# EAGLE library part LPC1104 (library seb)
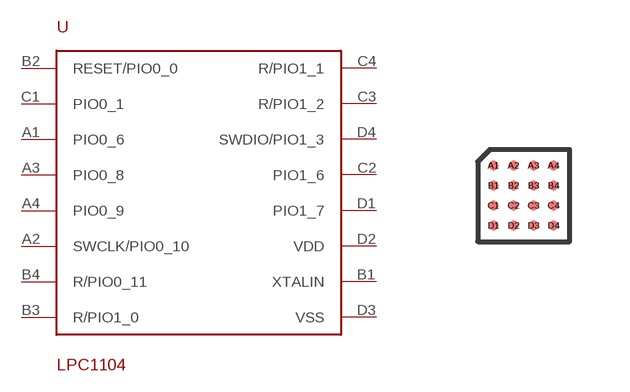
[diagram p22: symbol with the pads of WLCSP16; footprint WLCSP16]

Designator prefix -

## LPC1104  [WLCSP16]
A1  PIO0_6
A2  SWCLK/PIO0_10
A3  PIO0_8
A4  PIO0_9
B1  XTALIN
B2  RESET/PIO0_0
B3  R/PIO1_0
B4  R/PIO0_11
C1  PIO0_1
C2  PIO1_6
C3  R/PIO1_2
C4  R/PIO1_1
D1  PIO1_7
D2  VDD
D3  VSS
D4  SWDIO/PIO1_3

## Footprint WLCSP16 (pad centres in mm)
smd 0.25 x 0.25: A1 -0.75,0.75; A2 -0.25,0.75; A3 0.25,0.75; A4 0.75,0.75; B1 -0.75,0.25; B2 -0.25,0.25; B3 0.25,0.25; B4 0.75,0.25; C1 -0.75,-0.25; C2 -0.25,-0.25; C3 0.25,-0.25; C4 0.75,-0.25; D1 -0.75,-0.75; D2 -0.25,-0.75; D3 0.25,-0.75; D4 0.75,-0.75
